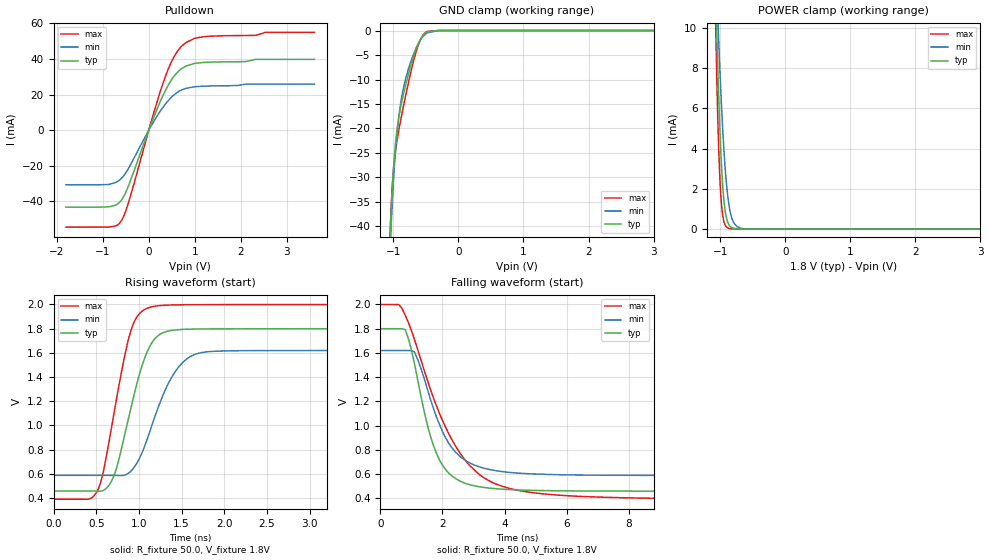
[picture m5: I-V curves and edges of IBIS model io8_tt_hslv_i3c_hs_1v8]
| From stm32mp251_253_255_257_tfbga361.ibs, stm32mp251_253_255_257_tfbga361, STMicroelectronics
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[Model]   io8_tt_hslv_i3c_hs_1v8
Model_type I/O_open_drain
Polarity   Non-Inverting
Enable   Active-Low
| CAP_THRESHOLD on pad IOTT is "UDTCAPC" :
| Rising=30.0% of vddiov33m   Falling=70.0% of vddiov33m
| C_comp min and max val. don't necessarily correlate with the min and max pvt
| but are the smallest and greatest pad capacitance found.
| var   typ   min   max
C_comp   1.23085pF  1.11693pF  1.38090pF
|C_comp_pulldown   1.23085pF  1.11693pF  1.38090pF
Vinl = 810.0mV
Vinh = 1.0V
Vmeas = 900.0mV   | Reference voltage for timing measurements
Cref  = 50.0pF   | Timing specification test load capacitance value
Rref  = 1.0MOhm   | Timing specification test load resistance value
Vref  = 990.0mV   | Timing specification test load voltage
[Model Spec]
| TIME_THRESHOLD on pin ZIV08M is "CMOS" :
| Rising=50.0% of vddv08m   Falling=50.0% of vddv08m
Vinl 675.70000mV 623.70000mV 735.70000mV
Vinh 1.12730V 1.01130V 1.24930V
| variable   typ   min   max
[Temperature Range] 25.0 125.0 -40.0
| variable   typ   min   max
[Voltage Range] 1.8V 1.62V 2.0V
| variable   typ   min   max
[POWER Clamp Reference] 1.8V 1.62V 2.0V
| variable   typ   min   max
[GND Clamp Reference] 0V 0V 0V
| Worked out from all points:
|   slope of the pulldown table from 0 to 0.27 V, typ, clamps not added: 15.6 ohm
|   GND clamp passes 1 mA (typ) near -0.55 V on its own axis
|   POWER clamp passes 1 mA (typ) near -0.93 V on its own axis
|   rising waveform, R_fixture 50.0, V_fixture 1.8V: 20-80 % time 287ps typ, 349ps min, 256ps max; typ from 0.458 V to 1.8 V
|   falling waveform, R_fixture 50.0, V_fixture 1.8V: 20-80 % time 805ps typ, 995ps min, 1.6ns max; typ from 1.8 V to 0.458 V
[POWER Clamp]
-1.8V     152.1mA    105.6mA    221.1mA
-1.07V    12.07mA    13.61mA    10.38mA
-1.05V    9.569mA    11.75mA    7.248mA
-1.03V    7.339mA    9.993mA    4.743mA
-1.01V    5.42mA     8.357mA    2.898mA
-990mV    3.841mA    6.859mA    1.662mA
-970mV    2.609mA    5.513mA    906.4uA
-940mV    1.358mA    3.806mA    344.1uA
-880mV    308.2uA    1.548mA    45.5uA
-790mV    28.46uA    298.8uA    2.106uA
-610mV    211.8nA    7.522uA    9.52nA
3.6V      0A         0A         0A
[GND Clamp]
-1.8V     -1.222A    -1.193A    -1.238A
-1.05V    -42.33mA   -45.55mA   -41.2mA
-1.04V    -38.89mA   -42.1mA    -37.88mA
-1.03V    -35.83mA   -38.98mA   -35.06mA
-1.01V    -30.7mA    -33.54mA   -30.61mA
-970mV    -23.47mA   -25.17mA   -24.97mA
-920mV    -18.06mA   -18.06mA   -20.63mA
-870mV    -14.51mA   -13.44mA   -17.13mA
-780mV    -9.532mA   -8.354mA   -11.38mA
-650mV    -3.743mA   -3.581mA   -4.327mA
-490mV    -324.1uA   -556uA     -259.6uA
3.6V      66.06nA    2.767uA    18.5nA
| variable   typ   min   max
[Pullup Reference] 1.8V 1.62V 2.0V
| variable   typ   min   max
[Pulldown Reference] 0V 0V 0V
[Pulldown]
-1.8V     -43.21mA   -30.64mA   -54.48mA
-870mV    -43.06mA   -30.5mA    -54.44mA
-700mV    -41.81mA   -29.1mA    -53.55mA
-600mV    -39.48mA   -27.21mA   -51.03mA
-440mV    -31.2mA    -21.48mA   -40.66mA
70mV      4.786mA    3.206mA    6.392mA
360mV     22.22mA    14.64mA    30.08mA
580mV     31.3mA     20.48mA    42.61mA
810mV     36.07mA    23.54mA    49.29mA
1.18V     38.05mA    24.73mA    52.5mA
2.54V     39.81mA    25.88mA    54.99mA
3.6V      39.81mA    25.88mA    54.99mA
[Ramp]
dV/dt_r 805.0234mV/286.21385ps 619.12346mV/348.29334ps 965.58598mV/255.6256ps
dV/dt_f 805.07299mV/802.41806ps 619.18344mV/992.29934ps 965.6265mV/1.59427ns
R_load = 50.0
| Removed startup time: 0s 0s 0s  .
| Removed end time: 6.975ns.
[Rising Waveform]
R_fixture   = 50.0
V_fixture   = 1.8V
V_fixture_min = 1.62V
V_fixture_max = 2.0V
0s        458.2mV    588mV      390.6mV
425ps     458.2mV    588mV      393.3mV
525ps     456.8mV    588mV      476.1mV
700ps     571.4mV    587.7mV    1.068V
900ps     1.125V     618.8mV    1.77V
1ns       1.409V     719.3mV    1.92V
1.125ns   1.651V     945.8mV    1.976V
1.425ns   1.789V     1.445V     1.997V
1.75ns    1.798V     1.604V     1.999V
6.975ns   1.8V       1.62V      2V
| Removed startup time: 0s 0s 0s  .
| Removed end time: 199.9ns.
[Falling Waveform]
R_fixture   = 50.0
V_fixture   = 1.8V
V_fixture_min = 1.62V
V_fixture_max = 2.0V
0s        1.8V       1.62V      2V
600ps     1.8V       1.62V      1.998V
800ps     1.792V     1.62V      1.913V
1.1ns     1.51V      1.608V     1.71V
1.7ns     842.5mV    1.149V     1.236V
2.3ns     584mV      818.5mV    885.4mV
2.9ns     510.1mV    688.6mV    663.5mV
3.8ns     476.7mV    624.2mV    509.5mV
7.1ns     459.1mV    589.9mV    408.5mV
199.9ns   458.2mV    588mV      390.6mV
